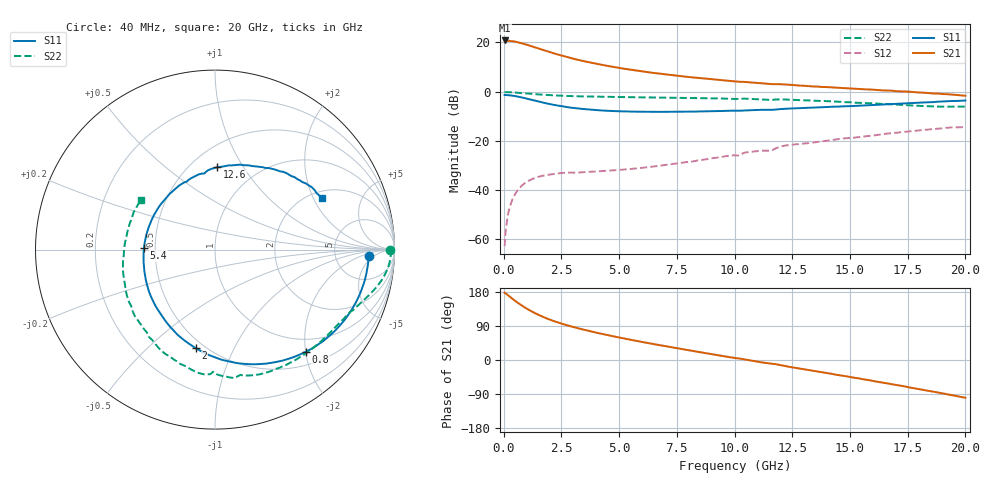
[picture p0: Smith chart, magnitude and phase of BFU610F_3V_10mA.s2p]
! Filename:  P:\Prog\Test\Noise\ATS_data\Testdata_Net\SplitFiles\BFU610_2W_A5_HighFreq_3V_10mA_D.s2p
! Date/Time: Wed 10/Aug/2011 16:57:27
! BFU610_2W_A5_HighFreq_3V_1mA_10mA_Bias4_R.s2p
! MDIF S-parameter v. bias file
! BFU610_2W_A5_HighFreq_3V_1mA_10mA
! Date/time Mon Aug 08 14:07:26 2011
! VAR V_out= 3.0000
! VAR I_out= 10.0000
! VAR V_in= 0.9181
! VAR I_in= 0.0933
! Device data file deembeded for feedlines and parallel
! Original file: \SplitFiles\BFU610_2W_A5_HighFreq_3V_10mA_R.s2p
! Feed-files: PR003V01_101208_Feed1.s2p, PR003V01_101208_Feed2.s2p
! Parallel-file: PR003V01_101208_Par.s2p
# MHz S MA R 50
!  Freq-MHz  S11-mag  S11-arg  S21-mag  S21-arg  S12-mag  S12-arg  S22-mag  S22-arg
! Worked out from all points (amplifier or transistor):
!   167 points, 40 MHz to 20 GHz, reference 50 ohm
!   highest |S21| = 20.8 dB at 40 MHz (marker M1)
!   |S21| within 3 dB of that: start of sweep to 1.425 GHz
!   unconditionally stable (mu >= 1): 2.534 GHz to end of sweep
!   at 550 MHz: K = 0.23, MSG = 30.5 dB, |S12| = -40.8 dB
!   at 4.2 GHz: K = 1.67, MAG = 16.8 dB, |S12| = -32.3 dB
!   at 20 GHz: K = 1.30, MAG = 3.1 dB, |S12| = -14.4 dB
!   S11 on the Smith chart (normalised r, x): 40 MHz: 12, -3; 800 MHz: 0.74, -2.01; 2 GHz: 0.45, -0.72; 5.4 GHz: 0.43, +0.01; 12.6 GHz: 0.67, +0.77; 20 GHz: 2.31, +2.34
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40  0.8571 -2.4  10.99 177.6  0.0007277 81.7  0.9771 -0.1
60  0.8556 -3.7  10.98 176.6  0.001165 90.1  0.9792 -0.5
140  0.854 -8.9  10.92 173.2  0.002404 83.9  0.9795 -2.0
360  0.834 -22.7  10.66 162.5  0.006152 78.3  0.9709 -5.5
550  0.8067 -34.3  10.27 153.7  0.0091 71.9  0.9579 -8.2
800  0.7618 -48.3  9.592 143.2  0.01251 64.2  0.9368 -11.4
1050  0.7136 -61.2  8.848 133.8  0.01522 57.6  0.9153 -14.1
1300  0.6673 -73.1  8.121 125.4  0.0173 52.3  0.895 -16.4
1650  0.6092 -87.8  7.191 115.2  0.01942 46.5  0.8707 -19.3
2000  0.5604 -100.9  6.38 106.5  0.02085 42.2  0.852 -21.9
2250  0.5317 -109.3  5.868 101.0  0.02139 40.4  0.8383 -23.9
2600  0.4976 -120.1  5.268 94.3  0.02245 37.7  0.8225 -26.0
3400  0.4471 -141.0  4.247 81.0  0.02302 36.3  0.803 -31.1
4300  0.4138 -160.9  3.478 68.3  0.02439 37.7  0.7884 -37.1
5400  0.3958 178.5  2.845 54.5  0.0267 41.7  0.7753 -44.7
6800  0.3896 156.1  2.307 38.6  0.03153 46.8  0.7602 -54.5
8800  0.4004 129.1  1.831 17.4  0.04262 50.4  0.7398 -69.3
10200  0.4104 112.4  1.591 4.0  0.05054 51.8  0.7142 -79.0
12600  0.4586 88.6  1.361 -20.4  0.08459 41.8  0.6812 -101.3
13400  0.4757 80.8  1.279 -28.3  0.09255 37.1  0.657 -109.2
16800  0.5613 51.9  1.05 -63.9  0.1432 13.7  0.5541 -152.2
20000  0.662 25.5  0.8279 -99.7  0.1916 -19.1  0.4978 146.2
